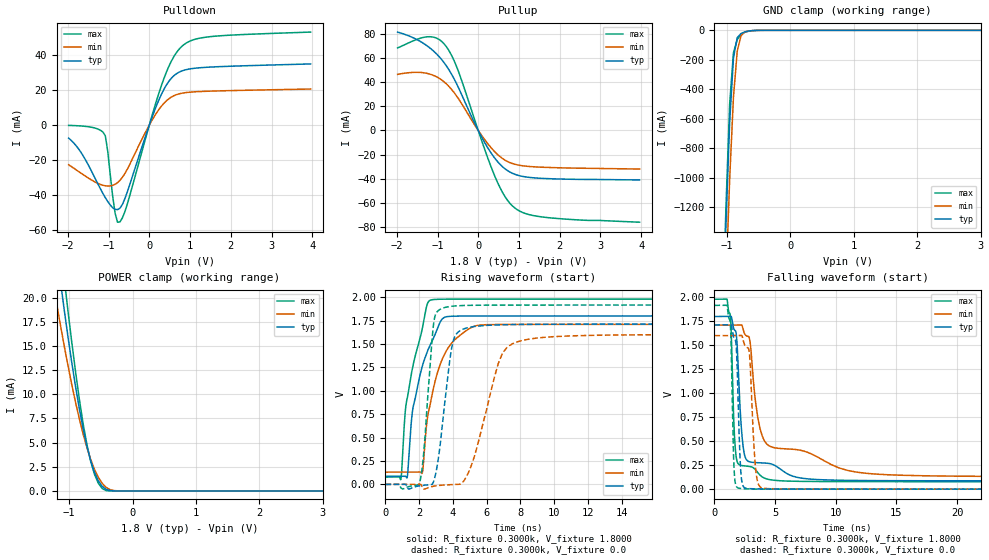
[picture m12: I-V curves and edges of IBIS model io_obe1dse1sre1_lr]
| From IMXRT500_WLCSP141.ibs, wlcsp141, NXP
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[Model] io_obe1dse1sre1_lr
|   Model io_obe1dse1sre1_lr
| Library cells for typ/min/max conditions are connected as defined below:
|  pad - External Pad
|  ipp_do - Core Input
|  ipp_obe - Output Buffer Enable
|  REFH3V3 - vdd1v8
|  gnde - gnde
|  ipp_dse - vdd
|  ipp_ina235_3v - NC
|  ipp_ina40_3v - NC
|  ipp_ina_mux - NC
|  ipp_ind - NC
|  ipp_ind_1p8v - NC
|  ipp_ind_3v - NC
|  ipp_sre - vdd
|  vdd - vdd
|  vdd1v8 - vdd1v8
|  vdda - vdde3v3
|  vdde3v3 - vdde3v3
| All other pins connected to ground
Model_type I/O
Polarity   Non-Inverting
Enable   Active-High
Vinl =   0.5400V
Vinh =   1.2600V
Vmeas =  0.9000V
Cref =   25.0000pF
Rref =   0.5000k
Vref =   0.0V
C_comp   2.2671pF   2.1738pF   2.3939pF
[Temperature Range]   25.0000   0.1250k   -40.0000
[Voltage Range]   1.8000V   1.7100V   1.9800V
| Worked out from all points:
|   slope of the pulldown table from 0 to 0.27 V, typ, clamps not added: 16.6 ohm
|   slope of the pullup table from 0 to 0.27 V, typ, clamps not added: 16.6 ohm
|   GND clamp passes 1 mA (typ) near -0.57 V on its own axis
|   POWER clamp passes 1 mA (typ) near -0.54 V on its own axis
|   rising waveform, R_fixture 0.3000k, V_fixture 1.8000: 20-80 % time 1.14ns typ, 1.17ns min, 1.05ns max; typ from 0.087 V to 1.8 V
|   rising waveform, R_fixture 0.3000k, V_fixture 0.0: 20-80 % time 660ps typ, 1.37ns min, 465ps max; typ from 0 V to 1.71 V
|   falling waveform, R_fixture 0.3000k, V_fixture 1.8000: 20-80 % time 490ps typ, 1.54ns min, 306ps max; typ from 1.8 V to 0.087 V
|   falling waveform, R_fixture 0.3000k, V_fixture 0.0: 20-80 % time 259ps typ, 370ps min, 195ps max; typ from 1.71 V to 0 V
[Pulldown]
|Voltage   I(typ)   I(min)   I(max)
-1.98V    -7.47mA    -22.75mA   -160uA
-1.62V    -17.76mA   -28.49mA   -590uA
-1.08V    -41.65mA   -34.85mA   -6.067mA
-840mV    -48.37mA   -34.01mA   -50.49mA
-780mV    -48.54mA   -33.06mA   -55.75mA
-720mV    -47.69mA   -31.71mA   -55.6mA
-540mV    -38.38mA   -25.32mA   -45.39mA
240mV     14.74mA    9.107mA    18.7mA
540mV     26.9mA     16.1mA     36.66mA
780mV     30.94mA    18.23mA    44.81mA
1.44V     33.27mA    19.47mA    50.67mA
3.96V     35.14mA    20.73mA    53.44mA
[Pullup]
|Voltage   I(typ)   I(min)   I(max)
-1.98V    81.32mA    46.37mA    68.19mA
-1.2V     68.55mA    46.7mA     77.5mA
-960mV    61.01mA    43.15mA    75.21mA
-780mV    53.26mA    38.46mA    69.13mA
-480mV    34.98mA    25.95mA    48.25mA
-60mV     4.085mA    3.083mA    6.056mA
240mV     -14.69mA   -11.22mA   -23.31mA
600mV     -30.11mA   -23.3mA    -51.48mA
900mV     -36.25mA   -27.97mA   -64.14mA
1.2V      -38.57mA   -29.61mA   -69.11mA
1.68V     -39.78mA   -30.54mA   -71.94mA
3.96V     -40.89mA   -31.89mA   -75.83mA
[GND_clamp]
|Voltage   I(typ)   I(min)   I(max)
-1.98V    -17.54A    -17.55A    -18.13A
-1.08V    -2.178A    -2.567A    -2.121A
-1.02V    -1.334A    -1.74A     -1.223A
-960mV    -626.1mA   -1.012A    -499.4mA
-900mV    -186.7mA   -452.2mA   -152mA
-840mV    -49.63mA   -139.9mA   -62.86mA
-780mV    -21.48mA   -35.54mA   -26.58mA
-720mV    -10.4mA    -11.15mA   -13.18mA
-600mV    -1.573mA   -2.152mA   -2.249mA
-480mV    -123.2uA   -243.9uA   -63.17uA
3.96V     0A         0A         0A
[POWER_clamp]
|Voltage   I(typ)   I(min)   I(max)
-1.98V    72.06mA    51.35mA    77.71mA
-1.26V    28.12mA    21.78mA    33.04mA
-1.2V     24.9mA     19.47mA    29.3mA
-1.14V    21.8mA     17.23mA    25.64mA
-1.08V    18.82mA    15.06mA    22.09mA
-1.02V    15.98mA    12.99mA    18.67mA
-840mV    8.51mA     7.462mA    9.493mA
-720mV    4.608mA    4.475mA    4.783mA
-600mV    1.908mA    2.218mA    1.702mA
-540mV    1.04mA     1.402mA    786.7uA
-420mV    173.6uA    383.7uA    43.39uA
3.96V     0A         0A         0A
[Ramp]
| variable   typ   min   max
dV/dt_r  0.7875/1.4045n   0.6809/2.9541n   0.9809/0.8116n
dV/dt_f  0.7773/6.0324n   0.5489/11.2378n   0.9301/3.1394n
R_load = 50.0000
[Rising Waveform]
R_fixture= 0.3000k
V_fixture= 1.8000
V_fixture_min= 1.7100
V_fixture_max= 1.9800
|time   V(typ)   V(min)   V(max)
0s        87.2mV     130.7mV    78.02mV
910.3ps   87.2mV     130.7mV    54.49mV
1.28ns    71.68mV    130.7mV    913.4mV
1.599ns   780.6mV    130.7mV    1.241V
2.179ns   1.26V      119.8mV    1.661V
2.507ns   1.432V     732.9mV    1.939V
3.299ns   1.751V     1.308V     1.978V
5.042ns   1.799V     1.672V     1.98V
7.144ns   1.8V       1.709V     1.98V
500ns     1.8V       1.71V      1.98V
[Rising Waveform]
R_fixture= 0.3000k
V_fixture= 0.0
V_fixture_min= 0.0
V_fixture_max= 0.0
|time   V(typ)   V(min)   V(max)
0s        10.47nV    703.5nV    40.19nV
2.028ns   -15.08mV   379.2uV    19.34mV
2.282ns   -9.27mV    -50.73mV   365.7mV
2.817ns   14.24mV    -20.84mV   1.658V
3.17ns    320.6mV    -11.21mV   1.863V
3.976ns   1.503V     -2.417mV   1.904V
4.911ns   1.675V     123.2mV    1.913V
7.235ns   1.707V     1.47V      1.916V
12.83ns   1.712V     1.594V     1.916V
500ns     1.712V     1.601V     1.916V
[Falling Waveform]
R_fixture= 0.3000k
V_fixture= 1.8000
V_fixture_min= 1.7100
V_fixture_max= 1.9800
|time   V(typ)   V(min)   V(max)
0s        1.8V       1.71V      1.98V
1.298ns   1.8V       1.71V      1.817V
1.632ns   1.663V     1.71V      597mV
1.889ns   1.46V      1.71V      281mV
2.212ns   649.6mV    1.712V     247.1mV
2.546ns   329.3mV    1.608V     241.7mV
3.936ns   273.8mV    556.4mV    127.9mV
6.184ns   149mV      417.9mV    83.69mV
23.11ns   87.27mV    133.1mV    78.02mV
500ns     87.2mV     130.7mV    78.02mV
[Falling Waveform]
R_fixture= 0.3000k
V_fixture= 0.0
V_fixture_min= 0.0
V_fixture_max= 0.0
|time   V(typ)   V(min)   V(max)
0s        1.712V     1.601V     1.916V
1.29ns    1.712V     1.601V     1.748V
1.568ns   1.592V     1.601V     366.2mV
1.749ns   1.541V     1.601V     46.58mV
2.188ns   155mV      1.602V     6.408mV
2.764ns   6.291mV    1.472V     2.463mV
2.908ns   5.181mV    1.376V     1.988mV
3.48ns    3.17mV     124.9mV    1.009mV
4.663ns   1.43mV     4.879mV    497.7uV
500ns     362.8nV    1.161uV    256.3nV
